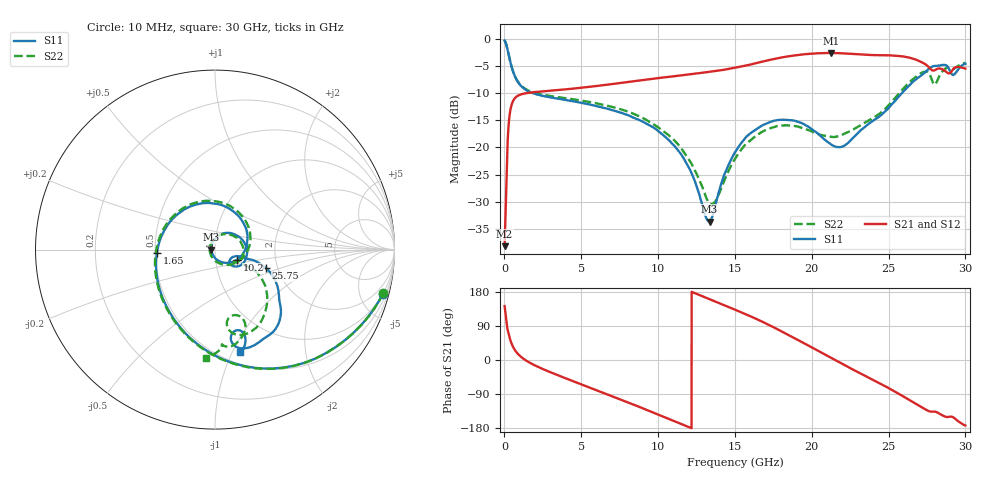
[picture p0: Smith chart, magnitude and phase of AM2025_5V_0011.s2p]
!Keysight Technologies,N5245B,MY58422270,A.16.20.02
!Date: Tuesday, July 14, 2026 01:03:06
!Correction: S11(C  2-Port  )
!S21(C  2-Port  )
!S12(C  2-Port  )
!S22(C  2-Port  )
!S2P File: Measurements: S11, S21, S12, S22:
# Hz S  dB  R 50
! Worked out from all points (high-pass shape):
!   3201 points, 10 MHz to 30 GHz, reference 50 ohm
!   highest |S21| = -2.59 dB at 21.25 GHz (marker M1); lowest = -38.2 dB at 10 MHz (marker M2)
!   |S21| within 3 dB of the highest: 14.47 GHz to 27.74 GHz (13.27 GHz wide, 62.9 % of centre); 29.2 GHz to end of sweep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
!   lowest |S11| = -33.7 dB at 13.35 GHz (marker M3), VSWR 1.04, Z = 48 + j0.014 ohm
!   |S11| at or under -10 dB: 1.852 GHz to 25.86 GHz (24.01 GHz wide, 173 % of centre)
!   |S22| runs from -30.5 to -0.3 dB; largest |S21 - S12| = 0.0057
!   S11 on the Smith chart (normalised r, x): 10 MHz: 1.00, -7.65; 1.65 GHz: 0.51, -0.02; 10.2 GHz: 1.27, -0.15; 25.75 GHz: 1.74, -0.40; 30 GHz: 0.61, -1.07
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1e7  -0.29 -14.7  -38.22 142.3  -40.58 162.0  -0.28 -14.5
2.536688e8  -2.63 -63.6  -16.55 72.1  -16.52 72.0  -2.63 -64.0
4.129906e8  -4.58 -90.0  -12.73 48.9  -12.72 48.9  -4.57 -90.5
8.159812e8  -7.66 -131.3  -10.57 18.8  -10.57 18.8  -7.60 -131.9
1.650078e9  -9.78 -176.7  -9.90 -7.2  -9.89 -7.2  -9.62 -177.2
5.014581e9  -11.79 91.0  -8.99 -64.4  -8.99 -64.4  -11.36 90.6
7.573103e9  -13.59 34.5  -8.11 -104.4  -8.11 -104.4  -12.97 33.5
1.000979e10  -16.97 -20.6  -7.23 -143.9  -7.23 -143.9  -16.30 -21.5
1.019723e10  -17.41 -25.3  -7.15 -147.0  -7.15 -147.1  -16.69 -25.9
1.183731e10  -22.85 -67.1  -6.59 -174.3  -6.60 -174.4  -21.54 -69.5
1.334618e10  -33.67 179.6  -6.05 160.5  -6.06 160.5  -30.29 -160.2
1.5005e10  -20.91 69.6  -5.30 132.8  -5.30 132.8  -22.08 76.9
1.783531e10  -14.93 -2.6  -3.52 79.8  -3.52 79.7  -16.01 3.0
2.000958e10  -16.66 -39.8  -2.71 33.0  -2.70 33.0  -17.09 -30.0
2.124667e10  -19.42 -41.0  -2.59 5.8  -2.59 5.8  -18.04 -32.2
2.292423e10  -17.59 -15.8  -2.82 -30.4  -2.81 -30.5  -16.33 -27.2
2.500479e10  -12.72 -15.8  -3.02 -74.1  -3.02 -74.2  -12.21 -27.4
2.574517e10  -10.38 -20.1  -3.17 -91.1  -3.16 -91.1  -9.82 -33.5
2.725404e10  -6.47 -40.2  -4.43 -127.1  -4.42 -127.2  -6.11 -63.7
2.802253e10  -4.98 -57.6  -5.74 -136.2  -5.73 -136.2  -8.40 -73.7
2.897847e10  -5.76 -79.9  -6.33 -149.6  -6.31 -149.8  -5.33 -84.1
3e10  -4.58 -76.2  -5.47 -172.9  -5.45 -173.0  -4.38 -94.8
